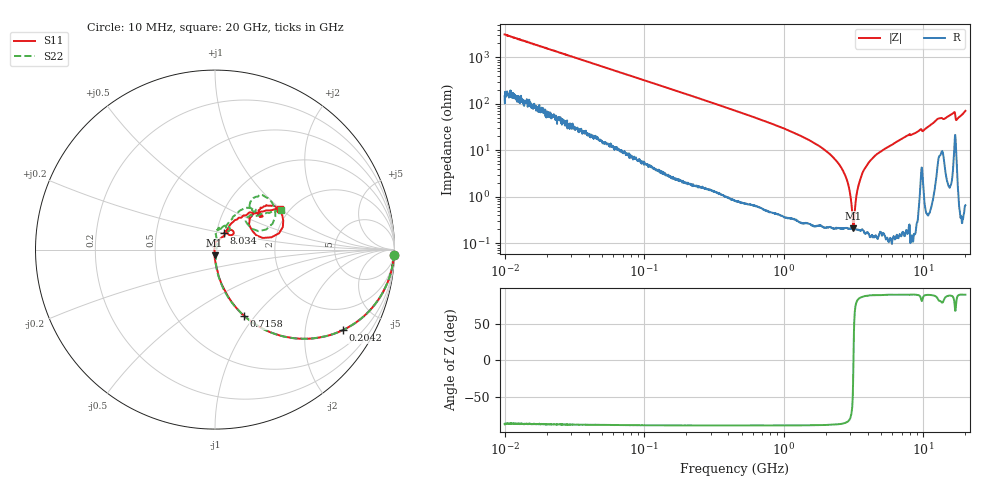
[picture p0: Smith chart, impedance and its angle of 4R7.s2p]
!Keysight Technologies,P5008B,MY61100088,A.16.20.02
!Date: Friday, August 30, 2024 13:01:43
!Correction: S11(C  2-Port  )
!S21(C  2-Port  )
!S12(C  2-Port  )
!S22(C  2-Port  )
!S2P File: Measurements: S11, S21, S12, S22:Log Frequency Sweep
# Hz S  dB  R 50
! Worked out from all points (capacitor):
!   1601 points, 10 MHz to 20 GHz, reference 50 ohm
!   read as one part in series: C = 5.09 pF near 10.39 MHz
!   lowest |Z| = 209 mohm at 3.151 GHz (marker M1)
!   series resonance near 3.156 GHz, so ESL is about 500 pH
!   S11 on the Smith chart (normalised r, x): 10 MHz: 3, -62; 204.2 MHz: 1.03, -3.16; 715.8 MHz: 1.00, -0.88; 8.034 GHz: 1.09, +0.20; 20 GHz: 1.78, +0.99
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1e7  -0.01 -1.8  -29.92 85.5  -29.92 85.5  -0.02 -1.8
3.555162e7  -0.08 -6.4  -19.11 81.9  -19.11 81.9  -0.08 -6.4
1.263918e8  -0.66 -21.4  -8.82 67.8  -8.83 67.8  -0.66 -21.4
2.042191e8  -1.50 -32.2  -5.53 57.1  -5.53 57.1  -1.50 -32.2
4.472136e8  -4.71 -54.3  -1.86 35.1  -1.87 35.1  -4.71 -54.3
7.15758e8  -7.91 -66.4  -0.81 23.0  -0.81 23.0  -7.91 -66.4
1.589917e9  -15.69 -81.1  -0.14 7.9  -0.14 7.9  -15.68 -81.5
2.496738e9  -22.67 -88.1  -0.04 1.4  -0.04 1.4  -22.55 -85.5
3.151135e9  -29.75 -94.8  -0.02 -1.9  -0.02 -1.9  -29.26 -81.1
3.416178e9  -34.44 -99.8  -0.01 -3.0  -0.02 -3.0  -33.38 -74.4
3.633803e9  -44.06 -110.1  -0.01 -3.9  -0.01 -3.9  -39.65 -53.1
3.774562e9  -44.79 172.9  -0.01 -4.5  -0.01 -4.5  -40.27 -11.4
3.958202e9  -41.36 107.2  -0.01 -5.2  -0.01 -5.2  -39.83 35.4
4.457348e9  -31.49 92.3  -0.01 -7.0  -0.01 -7.0  -31.39 66.5
5.652411e9  -26.33 76.5  -0.01 -11.0  -0.01 -11.0  -25.88 76.4
7.410252e9  -19.60 57.2  -0.03 -16.6  -0.04 -16.6  -19.67 85.0
8.03353e9  -19.53 61.6  -0.03 -18.3  -0.03 -18.4  -19.56 77.7
1.009107e10  -17.75 57.7  -0.13 -23.9  -0.13 -24.0  -17.57 62.9
1.291876e10  -10.02 38.0  -0.95 -34.7  -0.96 -34.8  -10.25 46.4
1.62275e10  -7.69 35.7  -0.99 -44.4  -0.99 -44.6  -7.82 46.1
1.767617e10  -11.75 42.5  -0.40 -42.6  -0.40 -42.8  -11.75 44.5
2e10  -7.40 32.1  -0.88 -57.4  -0.89 -57.6  -7.32 31.0
